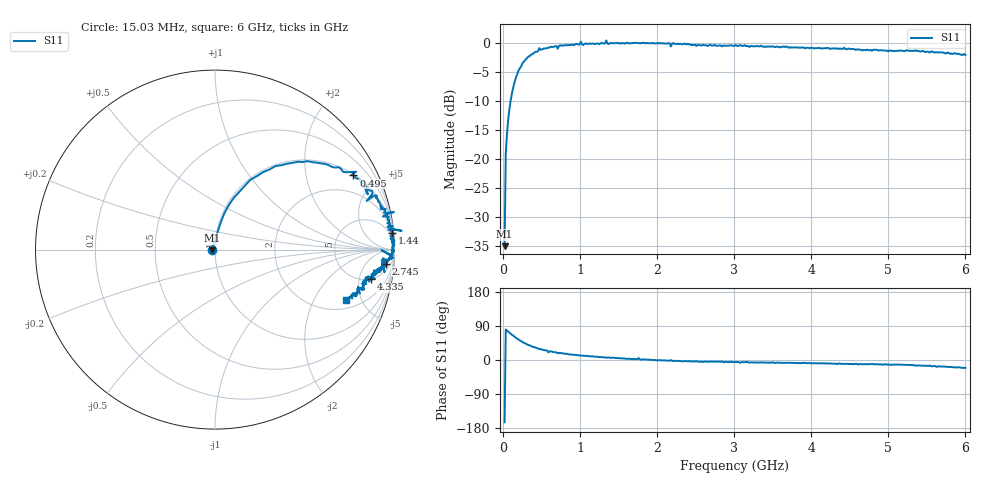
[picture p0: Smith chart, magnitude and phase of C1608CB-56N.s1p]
!	Network	Analyzer	HP8753E.07.74:	Oct	30	2002	Serial	No.	JP38451487
!	Hewlett-Packard
!	7	Sep	2009	9:47:04
!	Frequency	S11
#	HZ	S	RI	R	50
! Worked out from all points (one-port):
!   400 points, 15.03 MHz to 6 GHz, reference 50 ohm
!   lowest |S11| = -35.0 dB at 15.03 MHz (marker M1), VSWR 1.04, Z = 48.3 - j0.461 ohm
!   |S11| at or under -10 dB: start of sweep to 93.16 MHz
!   S11 on the Smith chart (normalised r, x): 15.03 MHz: 0.97, -0.01; 495 MHz: 1.05, +3.70; 1.44 GHz: 2, +21; 2.745 GHz: 10, -19; 4.335 GHz: 4.89, -7.48; 6 GHz: 2.58, -3.73
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1.502992e7  -0.0172 -0.00477
3.002985e7  0.018 0.109
6.00297e7  0.0536 0.206
1.050295e8  0.137 0.324
2.550287e8  0.467 0.49
4.650277e8  0.787 0.434
4.950275e8  0.771 0.413
5.850271e8  0.851 0.308
6.150269e8  0.85 0.359
7.650262e8  0.894 0.292
1.005025e9  0.997 0.209
1.035025e9  0.936 0.184
1.320023e9  0.98 0.118
1.335023e9  1.04 0.105
1.365023e9  0.966 0.112
1.440023e9  0.985 0.0936
1.515022e9  0.977 0.0768
1.755021e9  0.989 0.0863
2.145019e9  0.99 -0.0308
2.175019e9  0.928 -0.00351
2.265019e9  0.98 -0.0417
2.745016e9  0.954 -0.0785
3.015015e9  0.954 -0.0903
3.765011e9  0.9 -0.117
4.335008e9  0.87 -0.165
4.515007e9  0.87 -0.161
5.265004e9  0.831 -0.193
6e9  0.732 -0.279
